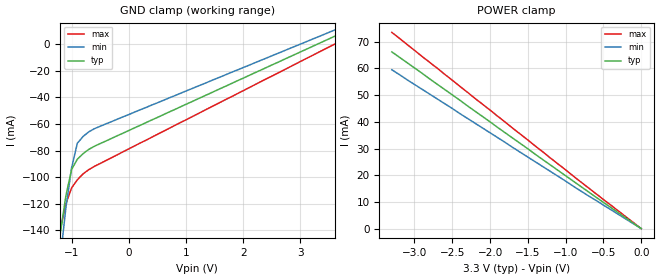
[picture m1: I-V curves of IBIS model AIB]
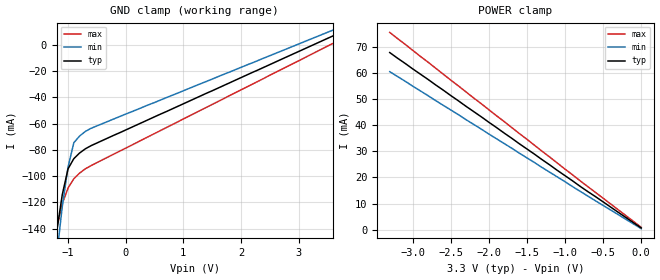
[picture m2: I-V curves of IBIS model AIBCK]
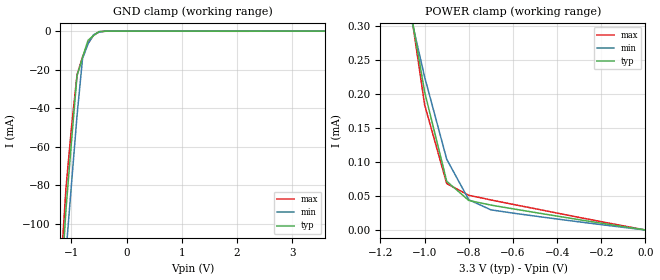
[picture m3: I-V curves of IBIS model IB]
|   Texas Instruments Incorporated
|   DVI group
|   IBIS Model for TFP401 REVN
|   100 pin PowerPAD Package
[IBIS Ver]   4.0
[Comment char]  |_char
[File name]   tfp401n_st1.ibs
[File Rev]   1.0
[Date]   6/10/2003
[Source]   File originated at Texas Instruments Incorporated.
   Connectivity Solutions Department. All data based on SPICE
   simulation.
[Notes]   File created by Ellen Yeh.
   PIN #3 (ST) set to high.
|Revision log: 1.0, 6/10/2003 Original release
[Disclaimer]
(C) Copyright Texas Instruments Incorporated 2003
   All rights reserved
  Texas Instruments Incorporated hereby grants the user of this IBIS
model a non-exclusive, nontransferable license to use this IBIS model
under the following terms.  Before using this IBIS model, the user
should read this license.  If the user does not accept these terms,
the IBIS model should be returned to Texas Instruments within 30 days.
  The user is granted this license only to use the IBIS model and
is not granted rights to sell, load, rent, lease or license the IBIS
model in whole or in part, or in modified form to anyone other than
user.  User may modify the IBIS model to suit its specific applications
but rights to derivative works and such modifications shall belong to
Texas Instruments.
  This IBIS model is provided on an "AS IS" basis and Texas Instruments
makes absolutely no warranty with respect to the information contained
herein.  TEXAS INSTRUMENTS DISCLAIMS AND CUSTOMER WAIVES ALL WARRANTIES,
EXPRESS OR IMPLIED, INCLUDING WARRANTIES OF MERCHANTABILITY OR FITNESS
FOR A PARTICULAR PURPOSE. The entire risk as to quality and performance
is with the Customer. ACCORDINGLY, IN NO EVENT SHALL THE COMPANY BE LIABLE
FOR ANY DAMAGES, WHETHER IN CONTRACT OR TORT,INCLUDING ANY LOST PROFITS
OR OTHER INCIDENTAL, CONSEQUENTIAL, EXEMPLARY, OR PUNITIVE DAMAGES ARISING
OUT OF THE USE OR APPLICATION OF THE IBIS model provided in this package.
Further, Texas Instruments reserves the right to discontinue or make changes
without notice to any product herein to improve reliability, function, or
design. Texas Instruments does not convey any license under patent rights
or any other intellectual property rights, including those of third parties.
IBIS Open Forum disclaims all warranties. See DISCLAIM.TXT
in vhdl.org:/pub/IBIS/models for the full disclaimer.
[Copyright]   Copyright 2003, Texas Instruments, All Rights Reserved
[Component]   TFP401
[Manufacturer]  Texas Instruments Incorporated
[Package]
|   typ   min   max
R_pkg   0.051   0.049   0.054
L_pkg   2.9nH   2.7nH   3.2nH
C_pkg   0.44pF   0.36pF   0.5pF
[Pin]   signal_name   model_name   R_pin   L_pin   C_pin
1   DFO   IOBOD
2   PDZ   IBPU
3   ST   IB
4   PIXS   IB
5   GND   GND
6   DVDD   POWER
7   STAG   IBF
8   SCDT   IOB
9   PDOZ   IBPU
10   QE0   OB
11   QE1   OB
12   QE2   OB
13   QE3   OB
14   QE4   OB
15   QE5   OB
16   QE6   OB
17   QE7   OB
18   OVDD   POWER
19   OGND   GND
20   QE8   OB
21   QE9   OB
22   QE10   OB
23   QE11   OB
24   QE12   OB
25   QE13   OB
26   QE14   OB
27   QE15   OB
28   OGND   GND
29   OVDD   POWER
30   QE16   OB
31   QE17   OB
32   QE18   OB
33   QE19   OB
34   QE20   OB
35   QE21   OB
36   QE22   OB
37   QE23   OB
38   DVDD   POWER
39   GND   GND
40   CTL1   IOB
41   CTL2   IOB
42   CTL3   IOB
43   OVDD   POWER
44   ODCK   OB2
45   OGND   GND
46   DE   OB
47   VSYNC   OB
48   HSYNC   OB
49   QO0   OB
50   QO1   OB
51   QO2   OB
52   QO3   OB
53   QO4   OB
54   QO5   OB
55   QO6   OB
56   QO7   OB
57   OVDD   POWER
58   OGND   GND
59   QO8   OB
60   QO9   OB
61   QO10   OB
62   QO11   OB
63   QO12   OB
64   QO13   OB
65	QO14   OB
66	QO15   OB
67	DVDD   POWER
68	GND   GND
69	QO16   OB
70	QO17		OB
71	QO18   OB
72	QO19   OB
73	QO20   OB
74	QO21   OB
75	QO22   OB
76	OGND   GND
77	QO23   OB
78	OVDD   POWER
79	AGND   GND
80	RX2+   AIB
81	RX2-		AIB
82	AVDD		POWER
83	AGND		GND
84	AVDD		POWER
85	RX1+		AIB
86	RX1-		AIB
87	AGND		GND
88	AVDD		POWER
89	AGND		GND
90	RX0+		AIB
91	RX0-		AIB
92	AGND		GND
93	RXC+		AIB
94	RXC-		AIBCK
95	AVDD		POWER
96	EXT_RES		AIB
97	PVDD		POWER
98	PGND		GND
99	RSVD		IBPU
100	OCK_INV		IB
| Models and submodels in the file (9): AIB (Input), AIBCK (Input), IB (Input), IBPU (Input), IBF (Input), IOB (I/O), IOBOD (I/O_open_sink), OB (3-state), OB2 (3-state)
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|   INPUT  MODEL
[Model]   AIB
Model_type   Input
| Signals   RX inputs
| variable   typ   min   max
C_comp   2pF   NA   NA
|   typ   min   max
[Temperature Range] 25.0   70.0   0.0
[Voltage range]   3.3V   3.0V   3.6V
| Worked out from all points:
|   POWER clamp passes 1 mA (typ) near -0.05 V on its own axis
[GND_clamp]
|Voltage   I(typ)   I(min)   I(max)
-3.6V     -1.3A      -1.32A     -1.29A
-1.2V     -143mA     -162mA     -140mA
-1.1V     -114mA     -123mA     -120mA
-1V       -94.2mA    -93mA      -108mA
-900mV    -86.5mA    -74.5mA    -102mA
-800mV    -82.3mA    -69.4mA    -97.5mA
-700mV    -79.1mA    -65.9mA    -94.3mA
-400mV    -72.8mA    -59.9mA    -87.5mA
3.6V      5.9mA      10.6mA     1.16nA
[Power_clamp]
|Note that the [Power_clamp] voltage table is referenced to Vcc
|and is calculated using Vtable=Vcc-Vmeasured.
|Voltage   I(typ)   I(min)   I(max)
-3.3V     66.2mA     59.5mA     73.5mA
-1V       19.8mA     17.8mA     22mA
-900mV    17.8mA     15.9mA     19.7mA
0V        9.76pA     46.7pA     8.21pA
|   INPUT  MODEL
[Model]   AIBCK
Model_type   Input
| Signals   RXC-
| variable   typ   min   max
C_comp   2pF   NA   NA
|   typ   min   max
[Temperature Range] 25.0   70.0   0.0
[Voltage range]   3.3V   3.0V   3.6V
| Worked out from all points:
|   POWER clamp passes 1 mA (typ) near -0.01 V on its own axis
[GND_clamp]
|Voltage   I(typ)   I(min)   I(max)
-3.6V     -1.3A      -1.32A     -1.29A
-1.3V     -185mA     -205mA     -177mA
-1.2V     -143mA     -162mA     -140mA
-1.1V     -114mA     -123mA     -121mA
-1V       -94.4mA    -93.1mA    -109mA
-900mV    -86.7mA    -74.6mA    -102mA
-800mV    -82.4mA    -69.5mA    -97.7mA
-700mV    -79.2mA    -66mA      -94.4mA
-600mV    -76.8mA    -63.6mA    -92mA
0V        -64.9mA    -52.8mA    -78.7mA
3.6V      6.69mA     11.1mA     1mA
[Power_clamp]
|Note that the [Power_clamp] voltage table is referenced to Vcc
|and is calculated using Vtable=Vcc-Vmeasured.
|Voltage   I(typ)   I(min)   I(max)
-3.3V     67.7mA     60.4mA     75.4mA
-800mV    16.6mA     14.7mA     18.7mA
-600mV    12.7mA     11.1mA     14.3mA
0V        727uA      458uA      1mA
|   INPUT  MODEL
[Model]   IB
Model_type   Input
| Signals   ST, PIXS, OCK_INV
Vinl = 1.08
Vinh = 2.10
| variable   typ   min   max
C_comp   2pF   NA   NA
|   typ   min   max
[Temperature Range] 25.0   70.0   0.0
[Voltage range]   3.3V   3.0V   3.6V
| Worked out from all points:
|   GND clamp passes 1 mA (typ) near -0.54 V on its own axis
|   POWER clamp passes 1 mA (typ) near -1.37 V on its own axis
[GND_clamp]
|Voltage   I(typ)   I(min)   I(max)
-3.6V     -1.31A     -1.33A     -1.29A
-1.2V     -138mA     -161mA     -126mA
-1.1V     -92.5mA    -115mA     -81.5mA
-1V       -57.2mA    -79.3mA    -49.9mA
-900mV    -23.2mA    -44mA      -22.7mA
-800mV    -13.6mA    -14.2mA    -13.4mA
-700mV    -4.78mA    -6.61mA    -6.2mA
-600mV    -2.27mA    -1.86mA    -2.19mA
-500mV    -190uA     -498uA     -401uA
-300mV    -548nA     -2.69uA    -1.84uA
3.6V      15.1uA     24.8uA     101pA
[Power_clamp]
|Note that the [Power_clamp] voltage table is referenced to Vcc
|and is calculated using Vtable=Vcc-Vmeasured.
|Voltage   I(typ)   I(min)   I(max)
-3.3V     5.57mA     4.01mA     6.85mA
-1.1V     392uA      367uA      405uA
-1V       203uA      225uA      184uA
-900mV    71.6uA     104uA      68.2uA
-800mV    43.4uA     44.4uA     51uA
-700mV    36.6uA     29.6uA     44.2uA
0V        35.3pA     99.7pA     34.3pA
